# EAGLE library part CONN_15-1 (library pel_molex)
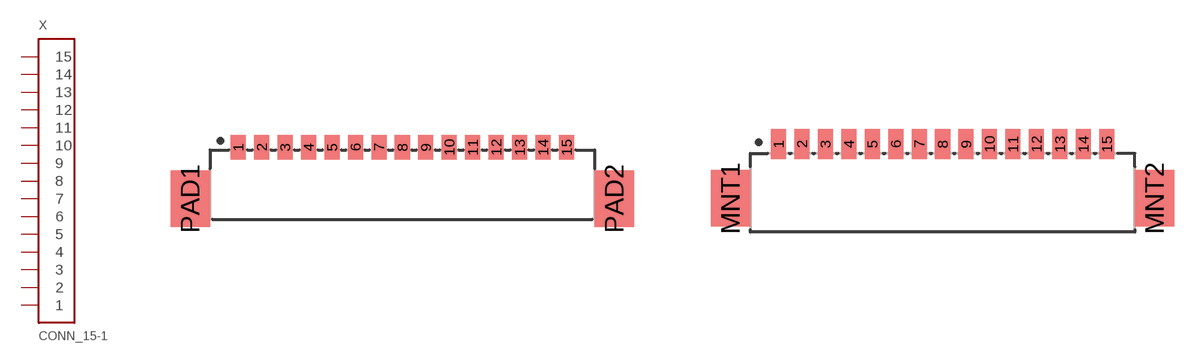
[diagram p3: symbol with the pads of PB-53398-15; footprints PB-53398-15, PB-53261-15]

Designator prefix X

## CONN_15-1-53398  [PB-53398-15]
1  1
2  2
3  3
4  4
5  5
6  6
7  7
8  8
9  9
10  10
11  11
12  12
13  13
14  14
15  15

## CONN_15-1-53261  [PB-53261-15]
Pads as for PB-53398-15

## CONN_15-1-53047  [PB-53047-15]
Pads as for PB-53398-15

## Footprint PB-53398-15 (pad centres in mm)
smd 0.8 x 1.3: 1 -8.75,1.25; 2 -7.5,1.25; 3 -6.25,1.25; 4 -5,1.25; 5 -3.75,1.25; 6 -2.5,1.25; 7 -1.25,1.25; 8 0,1.25; 9 1.25,1.25; 10 2.5,1.25; 11 3.75,1.25; 12 5,1.25; 13 6.25,1.25; 14 7.5,1.25; 15 8.75,1.25
smd 2.1 x 3: PAD1 -11.3,-1.5; PAD2 11.3,-1.5

## Footprint PB-53261-15 (pad centres in mm)
smd 0.8 x 1.6: 1 -8.75,1.1; 2 -7.5,1.1; 3 -6.25,1.1; 4 -5,1.1; 5 -3.75,1.1; 6 -2.5,1.1; 7 -1.25,1.1; 8 0,1.1; 9 1.25,1.1; 10 2.5,1.1; 11 3.75,1.1; 12 5,1.1; 13 6.25,1.1; 14 7.5,1.1; 15 8.75,1.1
smd 2.1 x 3: MNT1 -11.3,-1.8; MNT2 11.3,-1.8

## Footprint PB-53047-15 (pad centres in mm)
drill 0.5: 1 -8.75,0; 2 -7.5,0; 3 -6.25,0; 4 -5,0; 5 -3.75,0; 6 -2.5,0; 7 -1.25,0; 8 0,0; 9 1.25,0; 10 2.5,0; 11 3.75,0; 12 5,0; 13 6.25,0; 14 7.5,0; 15 8.75,0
